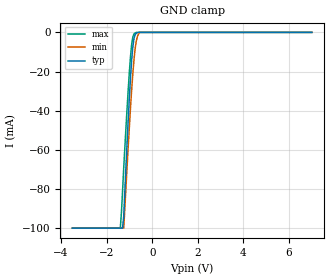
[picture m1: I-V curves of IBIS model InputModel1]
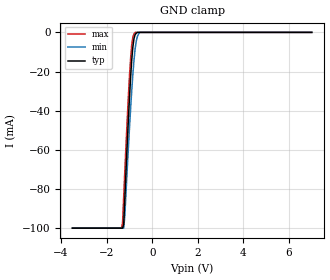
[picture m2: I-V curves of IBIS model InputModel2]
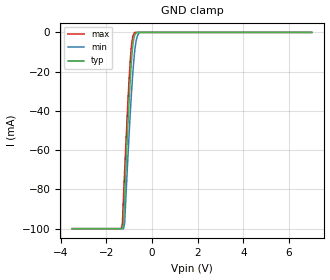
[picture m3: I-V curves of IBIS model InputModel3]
[IBIS Ver]   2.1
[File name]   pa200bl3.ibs   | pa= PSOP, f200bl= abbr chip name, 3= 3.3V Vcc
[File Rev]   2.00
[Date]   13-March-1996
[Source]   File generated from lab measurements at Intel Corporation
[Notes]   Rev 2.00 All data was replaced by actual measurements
   performed in a lab.
[Disclaimer] INTEL DEVELOPER'S SOFTWARE LICENSE AGREEMENT
| BY USING THIS SOFTWARE, YOU ARE AGREEING TO BE BOUND
| BY THE TERMS OFTHIS AGREEMENT.  DO NOT USE THE SOFTWARE
| UNTIL YOU HAVE CAREFULLY READAND AGREED TO THE FOLLOWING
| TERMS AND CONDITIONS.  IF YOU DO NOT AGREETO THE TERMS
| OF THIS AGREEMENT, PROMPTLY RETURN THE SOFTWARE PACKAGE
| ANDANY ACCOMPANYING ITEMS.
| IF YOU USE THIS SOFTWARE, YOU WILL BE BOUND BY THE TERMS
| OF THIS AGREEMENT
| LICENSE: Intel Corporation ("Intel") grants you the non-exclusive right
| to use the enclosed software program ("Software").  You will not use,
| copy, modify, rent, sell or transfer the Software or any portion
| thereof, except as provided in this Agreement.
| System OEM Developers may:
| 1.   Copy the Software for support, backup or archival purposes;
| 2.   Install, use, or distribute Intel owned Software in object code
|   only;
| 3.   Modify and/or use Software source code that Intel directly makes
|   available to you as an OEM Developer;
| 4.   Install, use, modify, distribute, and/or make or have made
|   derivatives ("Derivatives") of Intel owned Software under the
|   terms and conditions in this Agreement, ONLY if you are a System
|   OEM Developer and NOT an end-user.
| RESTRICTIONS:
| YOU WILL NOT:
| 1.   Copy the Software, in whole or in part, except as provided for
|   in this Agreement;
| 2.   Decompile or reverse engineer any Software provided in object
|   code format;
| 3.   Distribute any Software or Derivative code to any end-users,
|   unless approved by Intel in a prior writing.
| TRANSFER: You may transfer the Software to another OEM
| Developer if thereceiving party agrees to the terms of this
| Agreement at the sole risk of any receiving party.
| OWNERSHIP AND COPYRIGHT OF SOFTWARE:
| Title to the Software and all copies thereof remain with Intel
| or its vendors.  The Software iscopyrighted and is protected by
| United States and international copyright laws.  You will not
| remove the copyright notice from the Software.  You agree to
| prevent any unauthorized copying of the Software.
| DERIVATIVE WORK: OEM Developers that make or have made
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[Copyright]   Copyright 1996, Intel Corporation, All Rights Reserved
[Component]   E28F200BL   | 44-lead PSOP package, 28F200BL
[Manufacturer]  Intel   | Boot Block (tm)
|   | operating in 3.3V Vcc range
[Package]
|Variable   typ   min   max
R_pkg   145.5m   144.0m   147.0m
L_pkg   5.25nH   2.00nH   8.50nH
C_pkg   1.09pF   0.68pF   1.50pF
|***********************Pin Definition********************************
[Pin]   signal_name   model_name   R_pin   L_pin   C_pin
  1   VPP   POWER
  2   DU   InputModel6
  3   NC   InputModel1
  4   A7   InputModel1
  5   A6   InputModel1
  6   A5   InputModel1
  7   A4   InputModel1
  8   A3   InputModel1
  9   A2   InputModel1
 10   A1   InputModel1
 11   A0   InputModel2
 12   CE#   InputModel2
 13   GND   GND
 14   OE#   InputModel4
 15   DQ0   InputOutput1
 16   DQ8   InputOutput1
 17   DQ1   InputOutput1
 18   DQ9   InputOutput1
 19   DQ2   InputOutput1
 20   DQ10   InputOutput1
 21   DQ3   InputOutput1
 22   DQ11   InputOutput1
 23   VCC   POWER
 24   DQ4   InputOutput1
 25   DQ12   InputOutput1
 26   DQ5   InputOutput1
 27   DQ13   InputOutput1
 28   DQ6   InputOutput1
 29   DQ14   InputOutput1
 30   DQ7   InputOutput1
 31   DQ15   InputOutput2
 32   GND   GND
 33   BYTE#   InputModel2
 34   A16   InputModel2
 35   A15   InputModel1
 36   A14   InputModel1
 37   A13   InputModel1
 38   A12   InputModel1
 39   A11   InputModel1
 40   A10   InputModel1
 41   A9   InputModel1
 42   A8   InputModel1
 43   WE#   InputModel5
 44   RP#   InputModel3
|***********************Input Model 6******************************
[Model]   InputModel6
Model_type   Input
|   Model for DU and NC pins, excluding Pin #3.
Vinl = 0.8V
Vinh = 2.0V
|Variable   Typ   Min   Max
C_comp   5.61p   NA   7.6p
[Voltage Range]   3.3V   3.0V   3.6V
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| Models and submodels in the file (8): InputModel1 (Input), InputModel2 (Input), InputModel3 (Input), InputModel4 (Input), InputModel5 (Input), InputModel6 (Input), InputOutput1 (I/O), InputOutput2 (I/O)
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|*********************Input Model 1************************************
[Model]   InputModel1
Model_type   Input
|   Model for A[15:1] & NC (pin 3).
Vinl = 0.8V
Vinh = 2.0V
|Variable   Typ   Min   Max
C_comp   5.61p   NA   7.6p
[Voltage Range]   3.3V   3.0V   3.6V
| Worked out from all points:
|   GND clamp passes 1 mA (typ) near -0.74 V on its own axis
[GND_clamp]
|Voltage  I(typ)   I(min)   I(max)
-3.5V     -100mA     -100mA     -100mA
-1.4V     -100mA     -100mA     -100mA
-1.35V    -100mA     -100mA     -92.06mA
-1.3V     -100mA     -100mA     -81.04mA
-1.25V    -94.05mA   -100mA     -69.23mA
-1.1V     -55.84mA   -68.26mA   -38.39mA
-1V       -32.84mA   -47.78mA   -19.9mA
-900mV    -13.97mA   -29.09mA   -6.016mA
-800mV    -3.185mA   -14.07mA   -792.3uA
-700mV    -426.8uA   -4.481mA   0A
-550mV    0A         0A         0A
7V        0A         0A         0A
[Power_clamp]
| Input buffer circuits of this product do not intrinsically
| require a [Power_clamp] definition.  This zero current
| [Power_clamp] table is provided for the compatibility with
| some IBIS parsers.
|Voltage  I(typ)   I(min)   I(max)
-3.3V     0A         0A         0A
0V        0A         0A         0A
3.3V      0A         0A         0A
7V        0A         0A         0A
|*********************Input Model 2******************************
[Model]   InputModel2
Model_type   Input
|   Model for A[0], A[16], CE# & BYTE# pins.
Vinl = 0.8V
Vinh = 2.0V
|Variable   Typ   Min   Max
C_comp   5.61p   NA   7.6p
[Voltage Range]   3.3V   3.0V   3.6V
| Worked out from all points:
|   GND clamp passes 1 mA (typ) near -0.74 V on its own axis
[GND_clamp]
|Voltage  I(typ)   I(min)   I(max)
-3.5V     -100mA     -100mA     -100mA
-1.35V    -100mA     -100mA     -100mA
-1.3V     -100mA     -100mA     -97.31mA
-1.25V    -97.98mA   -100mA     -83.77mA
-1.2V     -84.29mA   -93.56mA   -70.52mA
-1.05V    -45.71mA   -60.05mA   -33.65mA
-950mV    -23.43mA   -39.44mA   -13.59mA
-850mV    -7.586mA   -21.73mA   -2.468mA
-750mV    -1.17mA    -8.517mA   0A
-650mV    0A         -2.085mA   0A
-550mV    0A         0A         0A
7V        0A         0A         0A
[Power_clamp]
| Input buffer circuits of this product do not intrinsically
| require a [Power_clamp] definition.  This zero current
| [Power_clamp] table is provided for the compatibility with
| some IBIS parsers.
|Voltage  I(typ)   I(min)   I(max)
-3.3V     0A         0A         0A
0V        0A         0A         0A
3.3V      0A         0A         0A
7V        0A         0A         0A
|***********************Input Model 3******************************
[Model]   InputModel3
Model_type   Input
|   Model for RP# pin.
Vinl = 0.8V
Vinh = 2.0V
|Variable   Typ   Min   Max
C_comp   5.61p   NA   7.6p
[Voltage Range]   3.3V   3.0V   3.6V
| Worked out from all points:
|   GND clamp passes 1 mA (typ) near -0.74 V on its own axis
[GND_clamp]
|Voltage  I(typ)   I(min)   I(max)
-3.5V     -100mA     -100mA     -100mA
-1.35V    -100mA     -100mA     -100mA
-1.3V     -100mA     -100mA     -97.77mA
-1.25V    -97.89mA   -100mA     -84.11mA
-1.2V     -84.17mA   -97.43mA   -70.88mA
-1.05V    -45.52mA   -62.23mA   -33.85mA
-950mV    -23.27mA   -40.65mA   -13.74mA
-850mV    -7.538mA   -22.21mA   -2.542mA
-750mV    -1.177mA   -8.633mA   0A
-650mV    0A         -2.115mA   0A
-550mV    0A         0A         0A
7V        0A         0A         0A
[Power_clamp]
| Input buffer circuits of this product do not intrinsically
| require a [Power_clamp] definition.  This zero current
| [Power_clamp] table is provided for the compatibility with
| some IBIS parsers.
|Voltage  I(typ)   I(min)   I(max)
-3.3V     0A         0A         0A
0V        0A         0A         0A
3.3V      0A         0A         0A
7V        0A         0A         0A
